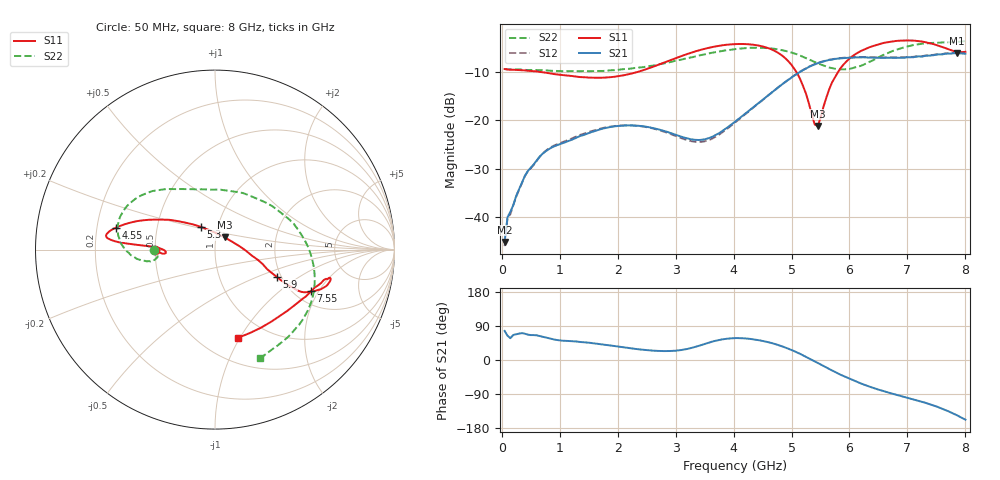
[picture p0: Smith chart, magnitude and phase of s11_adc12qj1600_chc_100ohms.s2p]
#  HZ  S  DB  R  100.00
! Rohde & Schwarz ZVA24 4Ports - Version 4.10 - 1145.1110k26 SN: 100644
! Date: 2020-07-21 15:24:56
! Measurements: S11 S31 S13 S33
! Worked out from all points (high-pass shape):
!   160 points, 50 MHz to 8 GHz, reference 100 ohm
!   highest |S21| = -6.17 dB at 7.85 GHz (marker M1); lowest = -45.2 dB at 50 MHz (marker M2)
!   |S21| within 3 dB of the highest: 5.277 GHz to end of sweep
!   lowest |S11| = -21.2 dB at 5.45 GHz (marker M3), VSWR 1.19, Z = 110 + j15.2 ohm
!   |S11| at or under -10 dB: 641.6 MHz to 2.359 GHz (1.717 GHz wide, 114 % of centre); 5.081 GHz to 5.807 GHz (726.2 MHz wide, 13.3 % of centre)
!   |S22| runs from -9.9 to -3.7 dB; largest |S21 - S12| = 0.014
!   S11 on the Smith chart (normalised r, x): 50 MHz: 0.50, -0.00; 4.55 GHz: 0.28, +0.10; 5.3 GHz: 0.83, +0.22; 5.9 GHz: 1.90, -0.67; 7.55 GHz: 2.44, -1.72; 8 GHz: 0.74, -0.98
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5e7  -9.46 -179.6  -45.21 76.7  -46.05 69.6  -9.43 179.9
1e8  -9.54 179.9  -40.08 64.1  -40.18 62.8  -9.52 179.7
4.5e8  -9.80 -178.1  -30.54 67.0  -30.60 67.0  -9.66 179.9
8e8  -10.29 -176.6  -26.10 57.6  -25.95 58.7  -9.76 -178.8
1.4e9  -11.12 -175.6  -23.13 47.0  -22.89 46.3  -9.88 -175.2
2.05e9  -10.85 -179.8  -21.17 34.5  -21.13 33.0  -9.54 -171.4
2.7e9  -8.57 177.0  -21.89 24.0  -22.01 22.2  -8.52 -170.2
3.45e9  -5.43 175.7  -24.07 39.8  -24.49 40.0  -6.54 -176.3
4.05e9  -4.28 173.2  -20.09 57.9  -20.28 59.2  -5.29 172.0
4.55e9  -4.94 167.6  -15.34 48.7  -15.37 50.2  -5.10 158.6
5e9  -8.60 153.3  -11.21 26.4  -11.17 27.6  -6.05 141.4
5.3e9  -16.55 121.6  -9.01 4.6  -8.96 5.8  -7.45 127.3
5.35e9  -18.87 106.9  -8.74 0.5  -8.69 1.7  -7.73 124.8
5.45e9  -21.23 51.9  -8.26 -7.5  -8.22 -6.2  -8.24 119.3
5.7e9  -12.20 -13.5  -7.49 -27.7  -7.43 -26.0  -9.26 102.4
5.9e9  -8.49 -23.8  -7.17 -42.5  -7.12 -40.8  -9.49 84.8
6.35e9  -4.92 -24.6  -7.07 -70.5  -7.00 -68.9  -7.93 36.9
6.7e9  -3.83 -19.0  -7.11 -87.2  -7.03 -85.8  -5.94 5.4
7.1e9  -3.56 -14.0  -7.01 -103.9  -6.94 -102.7  -4.49 -22.3
7.55e9  -4.68 -23.4  -6.42 -125.6  -6.35 -124.5  -3.99 -47.1
7.85e9  -5.86 -52.3  -6.17 -145.5  -6.09 -144.5  -3.85 -60.8
8e9  -5.89 -75.1  -6.29 -157.5  -6.21 -156.6  -3.67 -67.3
